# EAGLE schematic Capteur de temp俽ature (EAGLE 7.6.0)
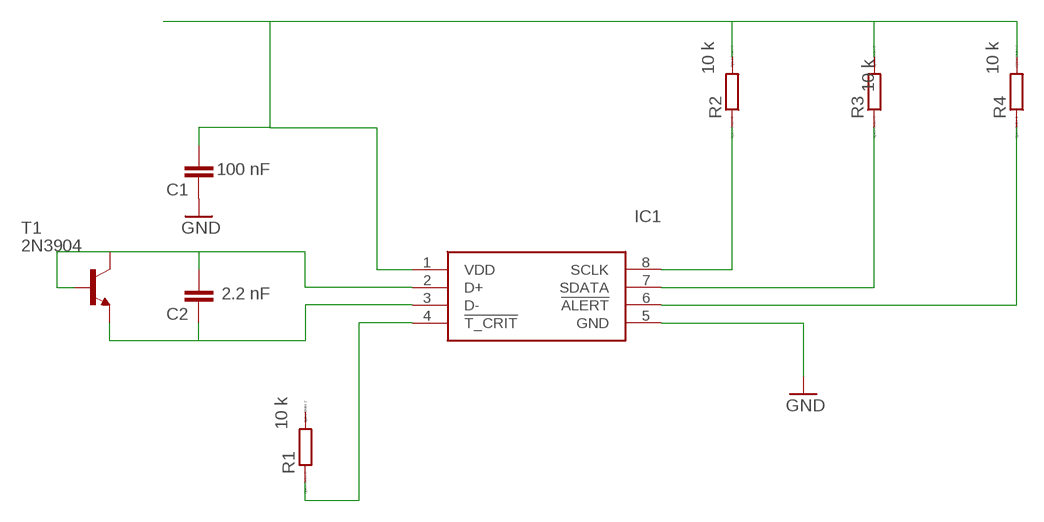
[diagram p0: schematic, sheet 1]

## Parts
C1  C2,5-3  [C2.5-3]
C2  C2,5-3  [C2.5-3]
IC1  SA56004AD,118  [SOIC127P600X175-8N]
R1  R  [R0805]
R2  R  [R0805]
R3  R  [R0805]
R4  R  [R0805]
T1  2N3904  [TO92]

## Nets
GND: C1.1 IC1.5(GND)
N$1: C1.2 IC1.1(VDD) R2.2 R3.2 R4.2
N$2: IC1.6(!ALERT) R4.1
N$3: IC1.7(SDATA) R3.1
N$4: IC1.8(SCLK) R2.1
N$5: C2.2 IC1.2(D+) T1.1(C) T1.2(B)
N$6: C2.1 IC1.3(D-) T1.3(E)
N$7: IC1.4(!T_CRIT) R1.1
Unconnected: R1.2

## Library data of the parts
C1 = capacitor-wima:C: CAPACITOR; C1: 100 nF
C2 = capacitor-wima:C: CAPACITOR; C2: 2.2 nF
IC1 = SA56004AD_118:SA56004AD,118: Board Mount Temperature Sensors I2C LOC +/- 2OC AND Source: Datasheet; ARROW_PART_NUMBER: SA56004AD,118; ARROW_PRICE-STOCK: https://www.arrow.com/en/products/sa56004ad118/nxp-semiconductors?region=nac; DESCRIPTION: Board Mount Temperature Sensors I2C LOC +/- 2OC AND; HEIGHT: 1.75mm; MANUFACTURER_NAME: NXP; MANUFACTURER_PART_NUMBER: SA56004AD,118; MOUSER_PART_NUMBER: 771-SA56004AD118; MOUSER_PRICE-STOCK: https://www.mouser.co.uk/ProductDetail/NXP-Semiconductors/SA56004AD118?qs=LOCUfHb8d9uULHX2Om8wPw%3D%3D
R1 = eagle-ltspice:R: RESISTOR, European symbol; R1: 10 k; SPICEMODEL: NONE; SPICEPREFIX: R
R2 = eagle-ltspice:R: RESISTOR, European symbol; R2: 10 k; SPICEMODEL: NONE; SPICEPREFIX: R
R3 = eagle-ltspice:R: RESISTOR, European symbol; R3: 10 k; SPICEMODEL: NONE; SPICEPREFIX: R
R4 = eagle-ltspice:R: RESISTOR, European symbol; R4: 10 k; SPICEMODEL: NONE; SPICEPREFIX: R
T1 = transistor:2N3904: NPN TRANSISTOR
